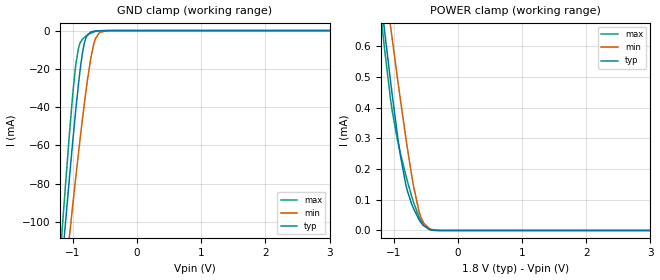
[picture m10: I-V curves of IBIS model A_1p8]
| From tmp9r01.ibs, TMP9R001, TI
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|   Model
[Model]   A_1p8
Model_type   Input
Vinl = 0.54
Vinh = 1.26
|   typ   min   max
C_comp   0.794pF   0.780pF   0.806pF
[Voltage Range]   1.8   1.7   2
[Temperature Range]   25   125   -40
[Power Clamp Reference]   1.8   1.7   2
[GND Clamp Reference]   0   0   0
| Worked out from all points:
|   GND clamp passes 1 mA (typ) near -0.73 V on its own axis
[GND Clamp]
|   Voltage   I(typ)   I(min)   I(max)
-1.8V     -380.2mA   -355.1mA   -412.2mA
-1.174V   -122.7mA   -145.4mA   -106.5mA
-1.147V   -112.1mA   -136.7mA   -94.11mA
-1.06V    -78.84mA   -109mA     -55.93mA
-1.001V   -56.95mA   -90.37mA   -32.33mA
-952.2mV  -40.06mA   -75.45mA   -16.84mA
-892.8mV  -21.71mA   -57.78mA   -6.862mA
-828mV    -7.401mA   -39.57mA   -3.751mA
-725.4mV  -835.3uA   -15.15mA   -1.403mA
-649.8mV  -212.6uA   -4.226mA   -460.9uA
-444.6mV  -2.253uA   -19.6uA    -3.32uA
3.6V      0A         0A         0A
[POWER Clamp]
|   Voltage   I(typ)   I(min)   I(max)
-1.8V     1.89mA     1.903mA    2.041mA
-1.195V   741.5uA    895.9uA    690.8uA
-1.157V   672.8uA    834.5uA    614.9uA
-1.147V   653.3uA    817uA      593.7uA
-1.044V   472.7uA    652.7uA    414.7uA
-903.6mV  251.8uA    434.6uA    256.5uA
-795.6mV  134.1uA    276.8uA    165.4uA
-693mV    71.06uA    144.4uA    91.79uA
-612mV    36.81uA    65.43uA    45.99uA
-536.4mV  15.46uA    24.05uA    17.48uA
-444.6mV  3.488uA    5.928uA    3.109uA
3.6V      0A         0A         0A
